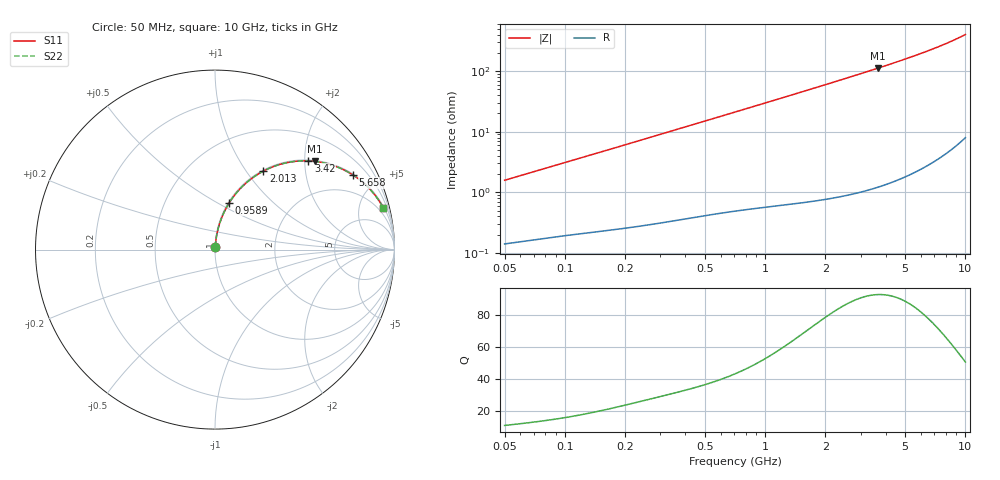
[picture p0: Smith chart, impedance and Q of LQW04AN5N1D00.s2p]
!Murata Part Number: LQW04AN5N1D00
!These Parameters are Measured in Series Mode Connection
!  o--[Z]--o
!Port1  Port2
!  o-------o
!Freq. Start=50[MHz] Stop=10[GHz], 401[Steps]
# Hz S RI R 50
!Freq.(Hz)	S 11(Real)	S 11(Imag)	S 21(Real)	S 21(Imag)	S 12(Real)	S 12(Imag)	S 22(Real)	S 22(Imag)
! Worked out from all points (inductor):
!   401 points, 50 MHz to 10 GHz, reference 50 ohm
!   read as one part in series: L = 4.97 nH near 51.34 MHz
!   highest Q = 92.4 at 3.654 GHz (marker M1), where L = 4.87 nH
!   S11 on the Smith chart (normalised r, x): 50 MHz: 1.00, +0.03; 958.9 MHz: 1.01, +0.57; 2.013 GHz: 1.02, +1.20; 3.42 GHz: 1.02, +2.09; 5.658 GHz: 1.04, +3.65; 10 GHz: 1.16, +8.07
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5e7  0.00165 0.0157  0.9984 -0.0157  0.9984 -0.0157  0.00165 0.0157
1.214486e8  0.00345 0.037  0.9966 -0.037  0.9966 -0.037  0.00345 0.037
1.956524e8  0.00601 0.0589  0.994 -0.0589  0.994 -0.0589  0.00601 0.0589
2.949953e8  0.0109 0.0878  0.9891 -0.0878  0.9891 -0.0878  0.0109 0.0878
4.689809e8  0.0231 0.1369  0.9769 -0.1369  0.9769 -0.1369  0.0231 0.1369
7.071068e8  0.0469 0.2002  0.9531 -0.2002  0.9531 -0.2002  0.0469 0.2002
9.589462e8  0.0797 0.2613  0.9203 -0.2613  0.9203 -0.2613  0.0797 0.2613
1.300479e9  0.1343 0.333  0.8657 -0.333  0.8657 -0.333  0.1343 0.333
1.504464e9  0.1709 0.3691  0.8291 -0.3691  0.8291 -0.3691  0.1709 0.3691
1.717543e9  0.2111 0.4013  0.7889 -0.4013  0.7889 -0.4013  0.2111 0.4013
2.013439e9  0.2686 0.4369  0.7314 -0.4369  0.7314 -0.4369  0.2686 0.4369
2.659148e9  0.392 0.4825  0.608 -0.4825  0.608 -0.4825  0.392 0.4825
3.035766e9  0.4586 0.4928  0.5414 -0.4928  0.5414 -0.4928  0.4586 0.4928
3.420121e9  0.5207 0.4942  0.4793 -0.4942  0.4793 -0.4942  0.5207 0.4942
3.654301e9  0.5555 0.4915  0.4445 -0.4915  0.4445 -0.4915  0.5555 0.4915
4.171863e9  0.6241 0.4789  0.3759 -0.4789  0.3759 -0.4789  0.6241 0.4789
4.826234e9  0.6958 0.4545  0.3042 -0.4545  0.3042 -0.4545  0.6958 0.4545
5.657692e9  0.7668 0.417  0.2332 -0.417  0.2332 -0.417  0.7668 0.417
6.54512e9  0.8234 0.375  0.1766 -0.375  0.1766 -0.375  0.8234 0.375
7.571744e9  0.8711 0.328  0.1289 -0.328  0.1289 -0.328  0.8711 0.328
8.759398e9  0.91 0.278  0.09 -0.278  0.09 -0.278  0.91 0.278
1e10  0.9381 0.2313  0.0619 -0.2313  0.0619 -0.2313  0.9381 0.2313
